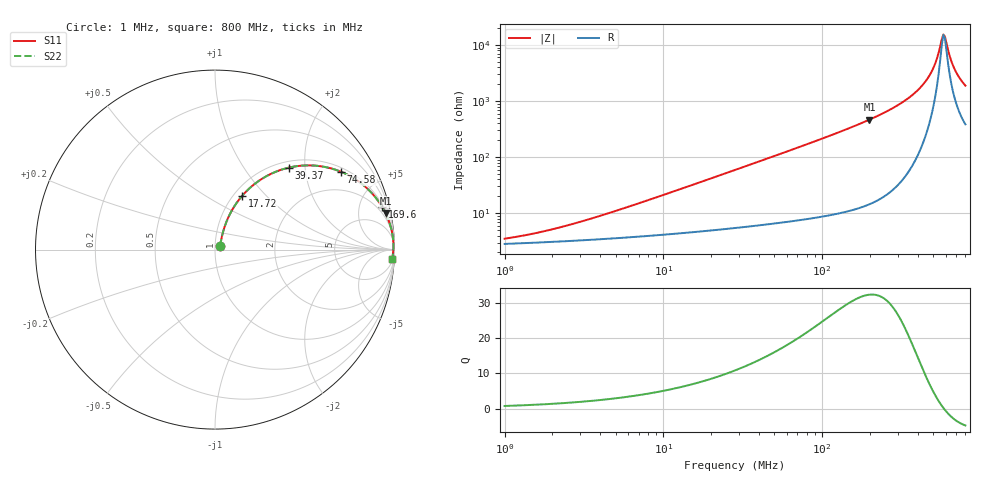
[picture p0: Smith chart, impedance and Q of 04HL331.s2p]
! Coilcraft 0402HL-331 Chip Inductor
! 20 July 2012
# MHz S MA R 50
!Freq  MagS11  AngS11  MagS21  AngS21  MagS12  AngS12  MagS22  AngS22
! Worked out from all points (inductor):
!   294 points, 1 MHz to 800 MHz, reference 50 ohm
!   read as one part in series: L = 330 nH near 5.288 MHz
!   highest Q = 32.3 at 198.9 MHz (marker M1), where L = 373 nH
!   self-resonance near 581.3 MHz
!   S11 on the Smith chart (normalised r, x): 1 MHz: 1.06, +0.04; 17.72 MHz: 1.10, +0.74; 39.37 MHz: 1.12, +1.64; 74.58 MHz: 1.15, +3.14; 169.6 MHz: 1.24, +7.68; 800 MHz: 9, -37
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1  0.03411 35.1  0.9723 -1.2  0.9723 -1.2  0.03411 35.1
1.729003  0.04547 47.9  0.9701 -2.0  0.9701 -2.0  0.04547 47.9
3.058438  0.069 59.1  0.9664 -3.5  0.9664 -3.5  0.069 59.1
9.354043  0.1872 67.6  0.9447 -10.6  0.9447 -10.6  0.1872 67.6
17.71853  0.334 63.3  0.9007 -19.3  0.9007 -19.3  0.334 63.3
28.60876  0.4932 55.3  0.826 -29.4  0.826 -29.4  0.4932 55.3
39.37434  0.6135 48.1  0.746 -37.7  0.746 -37.7  0.6135 48.1
74.58331  0.8262 31.6  0.5249 -55.6  0.5249 -55.6  0.8262 31.6
87.49813  0.8648 27.7  0.4656 -59.8  0.4656 -59.8  0.8648 27.7
169.5646  0.9603 14.5  0.25 -73.7  0.25 -73.7  0.9603 14.5
198.9264  0.9717 12.0  0.2082 -76.2  0.2082 -76.2  0.9717 12.0
267.6076  0.9854 8.1  0.1403 -80.0  0.1403 -80.0  0.9854 8.1
368.3093  0.9927 4.5  0.07846 -82.4  0.07846 -82.4  0.9927 4.5
452.2578  0.9944 2.4  0.04286 -81.2  0.04286 -81.2  0.9944 2.4
484.2956  0.9945 1.8  0.03153 -79.0  0.03153 -79.0  0.9945 1.8
518.603  0.9944 1.1  0.02054 -73.5  0.02054 -73.5  0.9944 1.1
581.2672  0.9937 0.1  0.006434 -10.1  0.006434 -10.1  0.9937 0.1
594.6808  0.9934 -0.1  0.007039 21.4  0.007039 21.4  0.9934 -0.1
636.8079  0.9926 -0.8  0.01554 61.3  0.01554 61.3  0.9926 -0.8
666.5377  0.992 -1.2  0.02257 68.5  0.02257 68.5  0.992 -1.2
713.7551  0.9907 -1.9  0.03354 73.0  0.03354 73.0  0.9907 -1.9
800  0.988 -2.9  0.05236 75.3  0.05236 75.3  0.988 -2.9
